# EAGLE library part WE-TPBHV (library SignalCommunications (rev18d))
WE-TPB HV Three-Phase Common Mode Power Line Choke Details see: http://katalog.we-online.de/en/pbs/WE-TPBHV Created by Yingchun Shan 2016 (C) Wurth Elektronik
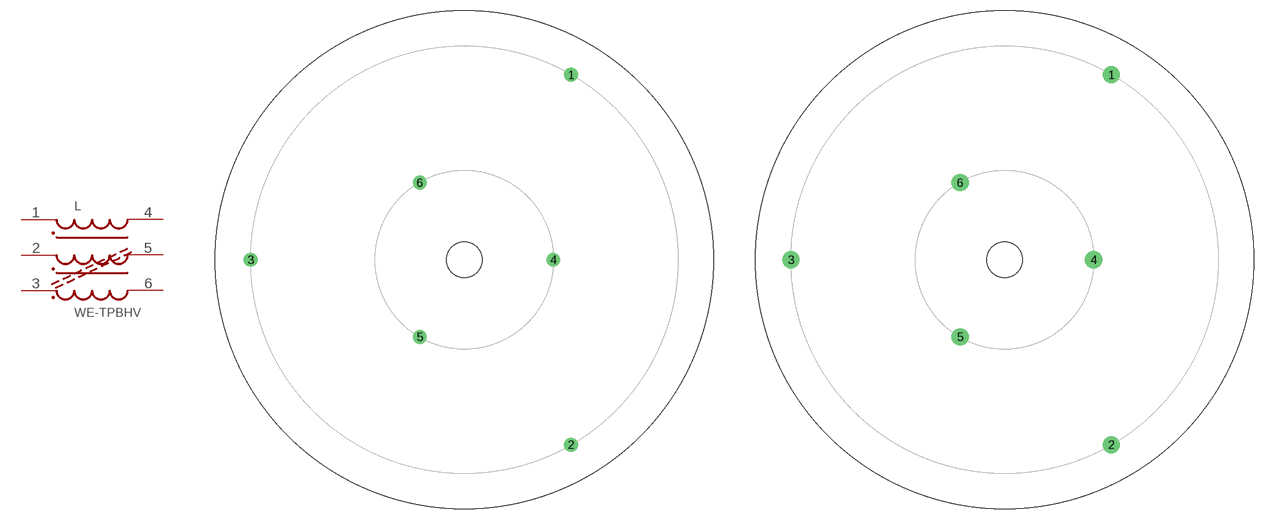
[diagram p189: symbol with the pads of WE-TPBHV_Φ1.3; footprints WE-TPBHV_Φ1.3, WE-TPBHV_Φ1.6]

Designator prefix L

## WE-TPBHV_744835150072  [WE-TPBHV_Φ1.3]
1  1  pas
2  2  pas
3  3  pas
4  4  pas
5  5  pas
6  6  pas

## WE-TPBHV_744839208072  [WE-TPBHV_Φ1.3]
Pads as for WE-TPBHV_Φ1.3

## WE-TPBHV_744835090095  [WE-TPBHV_Φ1.6]
Pads as for WE-TPBHV_Φ1.3

## WE-TPBHV_744838480095  [WE-TPBHV_Φ1.6]
Pads as for WE-TPBHV_Φ1.3

## WE-TPBHV_744839125095  [WE-TPBHV_Φ1.6]
Pads as for WE-TPBHV_Φ1.3

## WE-TPBHV_744835050135  [WE-TPBHV_Φ2.0]
Pads as for WE-TPBHV_Φ1.3

## WE-TPBHV_744835034160  [WE-TPBHV_Φ2.4]
Pads as for WE-TPBHV_Φ1.3

## WE-TPBHV_744838180160  [WE-TPBHV_Φ2.4]
Pads as for WE-TPBHV_Φ1.3

## WE-TPBHV_744839047160  [WE-TPBHV_Φ2.4]
Pads as for WE-TPBHV_Φ1.3

## WE-TPBHV_744835021220  [WE-TPBHV_Φ2.6]
Pads as for WE-TPBHV_Φ1.3

## WE-TPBHV_744837018220  [WE-TPBHV_Φ2.6]
Pads as for WE-TPBHV_Φ1.3

## WE-TPBHV_744839029220  [WE-TPBHV_Φ2.6]
Pads as for WE-TPBHV_Φ1.3

## WE-TPBHV_744837002460  [WE-TPBHV_Φ5.5]
Pads as for WE-TPBHV_Φ1.3

## WE-TPBHV_744838040400  [WE-TPBHV_Φ4.2]
Pads as for WE-TPBHV_Φ1.3

## WE-TPBHV_744839010400  [WE-TPBHV_Φ4.2]
Pads as for WE-TPBHV_Φ1.3

## WE-TPBHV_744839003460  [WE-TPBHV_Φ4.5]
Pads as for WE-TPBHV_Φ1.3

## WE-TPBHV_744837010290  [WE-TPBHV_Φ4.0]
Pads as for WE-TPBHV_Φ1.3

## WE-TPBHV_744837006400  [WE-TPBHV_Φ4.2]
Pads as for WE-TPBHV_Φ1.3

## Footprint WE-TPBHV_Φ1.3 (pad centres in mm)
drill 1.3: 1 15,25.981; 2 15,-25.981; 3 -30,0; 4 12.5,0; 5 -6.25,-10.825; 6 -6.25,10.825
hole 5 at 0,0

## Footprint WE-TPBHV_Φ1.6 (pad centres in mm)
drill 1.6: 1 15,25.981; 2 15,-25.981; 3 -30,0; 4 12.5,0; 5 -6.25,-10.825; 6 -6.25,10.825
hole 5 at 0,0

## Footprint WE-TPBHV_Φ2.0 (pad centres in mm)
drill 2: 1 15,25.981; 2 15,-25.981; 3 -30,0; 4 12.5,0; 5 -6.25,-10.825; 6 -6.25,10.825
hole 5 at 0,0

## Footprint WE-TPBHV_Φ2.4 (pad centres in mm)
drill 2.4: 1 15,25.981; 2 15,-25.981; 3 -30,0; 4 12.5,0; 5 -6.25,-10.825; 6 -6.25,10.825
hole 5 at 0,0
